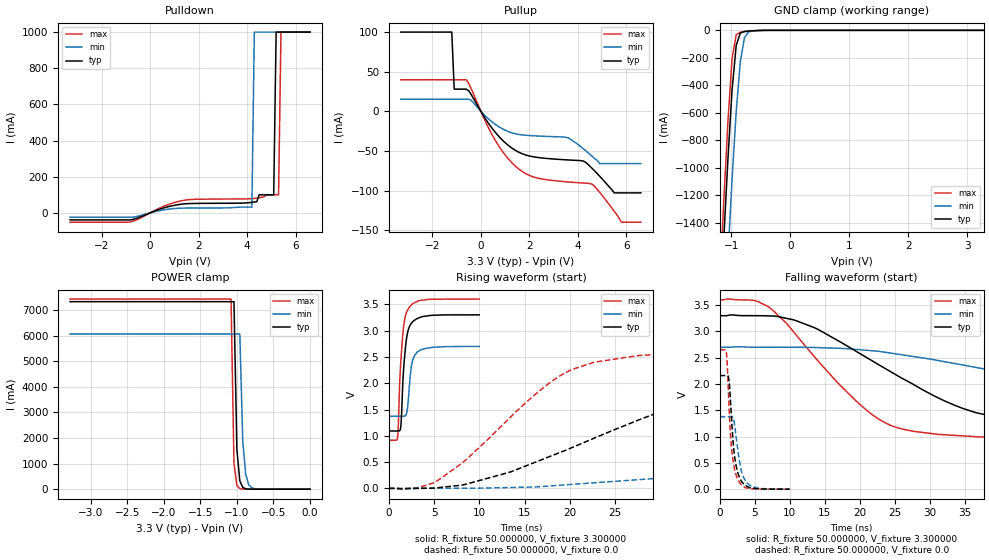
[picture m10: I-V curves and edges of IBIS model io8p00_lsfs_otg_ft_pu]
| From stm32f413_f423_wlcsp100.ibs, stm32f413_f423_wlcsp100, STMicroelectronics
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|   Model io8p00_lsfs_otg_ft_pu
[Model]  io8p00_lsfs_otg_ft_pu
Model_type I/O
Polarity   Non-Inverting
Enable   Active-Low
Vinl =   0.990000V
Vinh =   2.310000V
Vmeas =  1.650000V
Cref =   50.000000pF
Rref =   100.000000M
Vref =   0.0V
C_comp   8.196500pF   7.968500pF   8.492600pF
[Temperature Range]   25.000000   0.125000k   -40.000000
[Pullup Reference]   3.300000V   2.700000V   3.600000V
[Pulldown Reference]   0.0V   0.0V   0.0V
[POWER Clamp Reference]   3.300000V   2.700000V   3.600000V
[GND Clamp Reference]   0.0V   0.0V   0.0V
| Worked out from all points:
|   slope of the pulldown table from 0 to 0.495 V, typ, clamps not added: 20.1 ohm
|   slope of the pullup table from 0 to 0.495 V, typ, clamps not added: 21.8 ohm
|   GND clamp passes 1 mA (typ) near -0.52 V on its own axis
|   POWER clamp passes 1 mA (typ) near -0.80 V on its own axis
|   rising waveform, R_fixture 50.000000, V_fixture 3.300000: 20-80 % time 525ps typ, 500ps min, 526ps max; typ from 1.09 V to 3.3 V
|   rising waveform, R_fixture 50.000000, V_fixture 0.0: 20-80 % time 19.5ns typ, 47.4ns min, 10.3ns max; typ from 0.001 V to 2.16 V
|   falling waveform, R_fixture 50.000000, V_fixture 3.300000: 20-80 % time 18.3ns typ, 37.6ns min, 11.3ns max; typ from 3.3 V to 1.09 V
|   falling waveform, R_fixture 50.000000, V_fixture 0.0: 20-80 % time 845ps typ, 1.01ns min, 754ps max; typ from 2.16 V to 0.001 V
[Pulldown]
|Voltage   I(typ)   I(min)   I(max)
-3.3V     -38.65mA   -23.43mA   -51.3mA
-900mV    -38.65mA   -23.43mA   -51.3mA
1.4V      49.88mA    26.66mA    69.84mA
4.2V      58.43mA    32mA       78.86mA
4.3V      60.2mA     1A         80.13mA
4.4V      62mA       1A         81.72mA
4.5V      100mA      1A         83.79mA
5.1V      100mA      1A         100mA
5.2V      1A         1A         100mA
5.3V      1A         1A         100mA
5.4V      1A         1A         1A
6.6V      1A         1A         1A
[Pullup]
|Voltage   I(typ)   I(min)   I(max)
-3.3V     100mA      15.31mA    39.85mA
-1.2V     100mA      15.31mA    39.85mA
-1.1V     27.96mA    15.31mA    39.85mA
-600mV    27.96mA    15.31mA    39.85mA
500mV     -22.94mA   -14.36mA   -31.63mA
1.3V      -46.85mA   -27.39mA   -65.63mA
2.1V      -57.1mA    -30.77mA   -82.2mA
3.5V      -61.24mA   -32.7mA    -88.93mA
4.6V      -72.4mA    -57.1mA    -92.26mA
5.5V      -103mA     -66mA      -126.2mA
5.8V      -103mA     -66mA      -140mA
6.6V      -103mA     -66mA      -140mA
[GND_clamp]
|Voltage   I(typ)   I(min)   I(max)
-3.3V     -9.479A    -9.465A    -9.974A
-1.2V     -2.125A    -2.854A    -1.857A
-1.13V    -1.511A    -2.236A    -1.236A
-1.06V    -933.3mA   -1.641A    -660.9mA
-990mV    -433.3mA   -1.082A    -206.9mA
-920mV    -110.3mA   -591mA     -31.45mA
-850mV    -19.78mA   -226.7mA   -13.65mA
-780mV    -8.311mA   -53.93mA   -9.506mA
-710mV    -5.285mA   -11.94mA   -6.262mA
-640mV    -3.232mA   -4.282mA   -3.577mA
3.28V     0A         0A         0A
[POWER_clamp]
|Voltage   I(typ)   I(min)   I(max)
-3.28V    7.329A     6.064A     7.43A
-1.08V    7.329A     6.064A     7.43A
-1.04V    7.329A     6.064A     1.015A
-1V       1.545A     6.064A     138.8mA
-960mV    325.8mA    6.064A     19.13mA
-920mV    68.77mA    1.89A      2.772mA
-880mV    14.59mA    589.1mA    520.3uA
-840mV    3.154mA    183.6mA    196.4uA
-800mV    734.4uA    57.27mA    136.6uA
-720mV    96.98uA    5.605mA    116.7uA
0V        0A         0A         0A
[Ramp]
| variable   typ   min   max
dV/dt_r  1.29615/19.42797n   0.82720/47.34477n   1.59051/10.27092n
dV/dt_f  1.32486/18.27572n   0.79662/37.69738n   1.61078/11.28107n
R_load = 50.000000
[Rising Waveform]
R_fixture= 50.000000
V_fixture= 3.300000
V_fixture_min= 2.700000
V_fixture_max= 3.600000
|time   V(typ)   V(min)   V(max)
0s        1.092V     1.372V     915.2mV
940.9ps   1.092V     1.372V     944.8mV
1.061ns   1.092V     1.372V     1.265V
1.281ns   1.134V     1.372V     2.297V
1.662ns   2.352V     1.373V     3.123V
1.942ns   2.839V     1.412V     3.341V
2.222ns   3.055V     1.849V     3.438V
2.503ns   3.144V     2.341V     3.491V
3.163ns   3.232V     2.596V     3.557V
9.97ns    3.3V       2.7V       3.6V
[Rising Waveform]
R_fixture= 50.000000
V_fixture= 0.0
V_fixture_min= 0.0
V_fixture_max= 0.0
|time   V(typ)   V(min)   V(max)
0s        1.057mV    1.025mV    1.156mV
5.506ns   16.11mV    2.546mV    164.6mV
13.01ns   293.3mV    16.39mV    1.286V
20.02ns   762.8mV    74.66mV    2.245V
28.03ns   1.332V     173mV      2.532V
36.04ns   1.792V     308.6mV    2.603V
43.54ns   1.981V     446mV      2.628V
77.08ns   2.14V      1.055V     2.652V
105.1ns   2.159V     1.27V      2.652V
249.2ns   2.162V     1.38V      2.652V
[Falling Waveform]
R_fixture= 50.000000
V_fixture= 3.300000
V_fixture_min= 2.700000
V_fixture_max= 3.600000
|time   V(typ)   V(min)   V(max)
0s        3.3V       2.7V       3.6V
5.506ns   3.3V       2.7V       3.566V
11.01ns   3.199V     2.699V     2.915V
22.02ns   2.419V     2.63V      1.392V
31.03ns   1.745V     2.451V     1.044V
36.54ns   1.456V     2.316V     999.4mV
45.55ns   1.258V     2.102V     962.9mV
66.07ns   1.145V     1.673V     929mV
88.09ns   1.114V     1.504V     918.4mV
249.2ns   1.092V     1.372V     915.2mV
[Falling Waveform]
R_fixture= 50.000000
V_fixture= 0.0
V_fixture_min= 0.0
V_fixture_max= 0.0
|time   V(typ)   V(min)   V(max)
0s        2.162V     1.38V      2.652V
920.9ps   2.162V     1.38V      2.623V
1.041ns   2.164V     1.38V      2.462V
1.261ns   2.125V     1.379V     1.807V
1.702ns   1.322V     1.382V     767.4mV
2.102ns   644.9mV    1.246V     391.8mV
2.503ns   352.9mV    831.9mV    207.4mV
3.203ns   132.8mV    296mV      73.8mV
4.224ns   32.84mV    80.88mV    17.11mV
9.97ns    1.057mV    1.025mV    1.156mV
